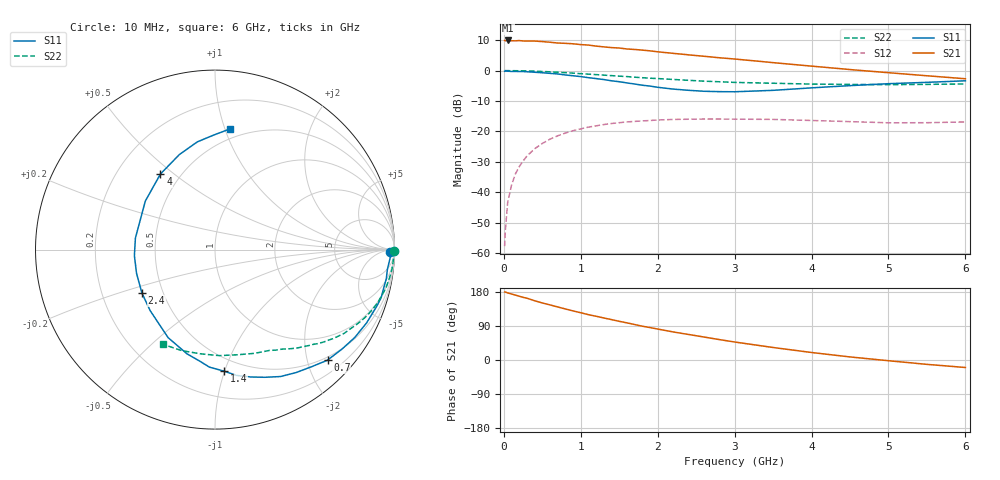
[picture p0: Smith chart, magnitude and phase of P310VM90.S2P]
! SIEMENS Small Signal Semiconductors
! BFP181
! Si NPN RF Bipolar Junction Transistor in SOT143
! VCE = 10 V  IC = 0.9 mA
! Common Emitter S-Parameters:  March  1996
# GHz  S  MA  R  50
!  f  S11  S21  S12  S22
! GHz  MAG  ANG  MAG  ANG  MAG  ANG  MAG  ANG
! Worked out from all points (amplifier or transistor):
!   36 points, 10 MHz to 6 GHz, reference 50 ohm
!   highest |S21| = 9.9 dB at 50 MHz (marker M1)
!   |S21| within 3 dB of that: start of sweep to 1.718 GHz
!   unconditionally stable (mu >= 1): 3.414 GHz to end of sweep
!   at 250 MHz: K = 0.08, MSG = 19.7 dB, |S12| = -29.7 dB
!   at 1.4 GHz: K = 0.47, MSG = 12.5 dB, |S12| = -17.4 dB
!   at 6 GHz: K = 1.30, MAG = 3.8 dB, |S12| = -16.9 dB
!   S11 on the Smith chart (normalised r, x): 10 MHz: 59, -31; 700 MHz: 0.44, -2.38; 1.4 GHz: 0.40, -0.99; 2.4 GHz: 0.38, -0.24; 4 GHz: 0.39, +0.45; 6 GHz: 0.42, +1.05
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0.01  0.9737 -0.8  3.119 179.4  0.0013 92.4  0.9974 -0.3
0.02  0.9811 -1.4  3.088 179.2  0.0024 85.9  0.9968 -0.6
0.05  0.9761 -3.0  3.123 177.1  0.0068 92.4  0.9958 -1.6
0.1  0.9668 -6.5  3.085 174.2  0.0131 84.4  0.9955 -3.1
0.15  0.9682 -9.6  3.078 171.3  0.02 82.6  0.9938 -4.7
0.2  0.964 -12.8  3.109 168.2  0.0263 80.8  0.9917 -6.3
0.25  0.9638 -16.1  3.063 165.3  0.0326 79.3  0.9882 -7.8
0.4  0.9382 -25.8  3.055 156.4  0.0518 72.9  0.9769 -12.3
0.5  0.9198 -32.2  2.992 150.5  0.0633 68.0  0.9646 -15.3
0.7  0.8789 -44.5  2.833 140.0  0.0847 60.3  0.9384 -20.8
0.9  0.821 -56.5  2.753 129.5  0.1028 52.6  0.907 -25.9
1.1  0.7635 -68.7  2.622 119.6  0.1176 46.0  0.8726 -30.5
1.4  0.6788 -85.8  2.383 106.6  0.1347 36.8  0.825 -36.9
1.8  0.574 -111.5  2.167 89.2  0.1488 27.1  0.7627 -43.7
2.2  0.4961 -136.7  1.919 74.1  0.1572 18.7  0.7144 -50.1
2.4  0.4738 -149.3  1.813 67.4  0.1585 15.1  0.6911 -53.1
3  0.4481 171.8  1.548 47.5  0.159 6.2  0.6386 -61.6
3.5  0.473 145.2  1.35 33.0  0.1574 1.0  0.6186 -69.1
4  0.5195 125.8  1.183 19.8  0.1512 -2.8  0.5993 -77.9
4.5  0.5653 110.6  1.038 8.1  0.1447 -5.1  0.5911 -87.7
5.5  0.6401 90.2  0.821 -11.5  0.139 -3.2  0.5926 -108.1
6  0.6788 82.7  0.733 -19.8  0.143 -2.1  0.602 -118.8
